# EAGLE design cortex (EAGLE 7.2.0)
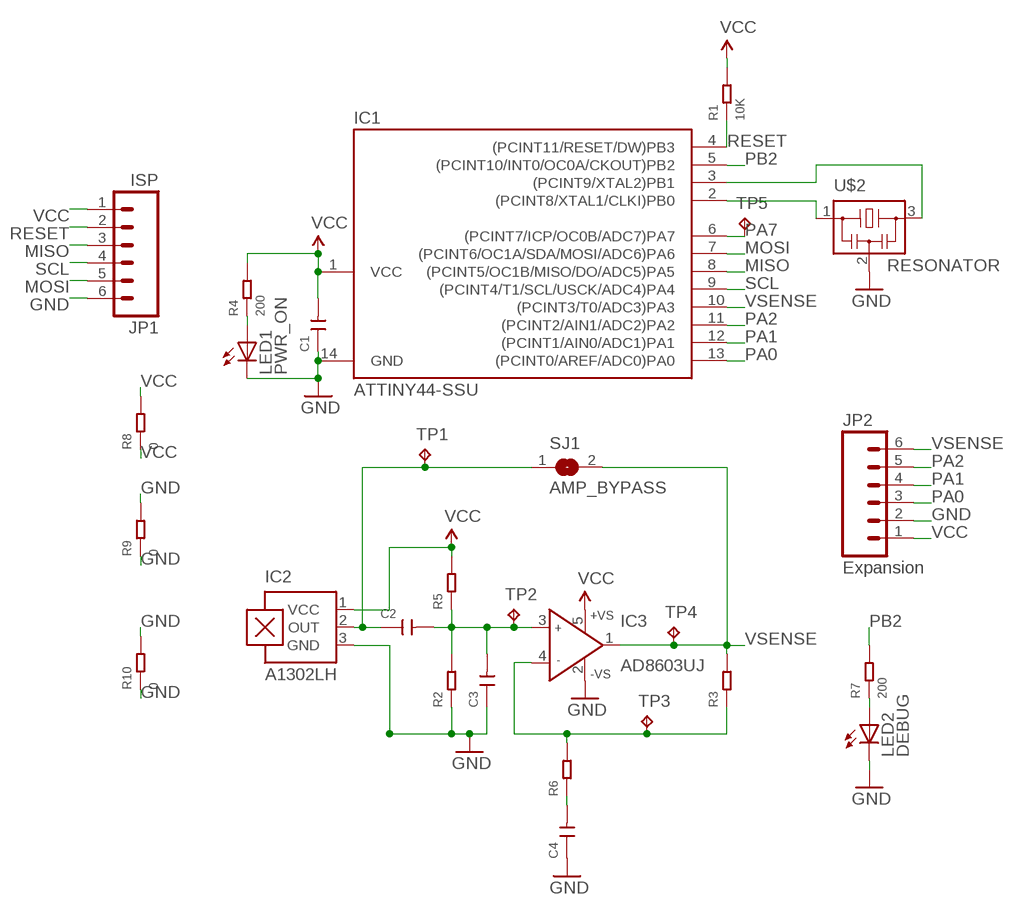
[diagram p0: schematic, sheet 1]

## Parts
C1  CAP-0805  [C0805]
C2  CAP-0805  [C0805]
C3  CAP-0805  [C0805]
C4  CAP-0805  [C0805]
IC1  ATTINY44-SSU  [SOIC14]
IC2  A1302LH  [SOT23-W]
IC3  AD8603UJ  [SOT23-5]
JP1  ISP  M06SMD-FEMALE-V2  [1X06-SMD-FEMALE-V2]
JP2  Expansion  M06SMD-FEMALE-V2  [1X06-SMD-FEMALE-V2]
LED1  PWR_ON  LEDCHIPLED_0805  [CHIPLED_0805]
LED2  DEBUG  LEDCHIPLED_0805  [CHIPLED_0805]
R1  10K  RES-0805  [R0805]
R2  RES-0805  [R0805]
R3  RES-0805  [R0805]
R4  200  RES-0805  [R0805]
R5  RES-0805  [R0805]
R6  RES-0805  [R0805]
R7  200  RES-0805  [R0805]
R8  0  RES-1206  [R1206]
R9  0  RES-1206  [R1206]
R10  0  RES-1206  [R1206]
SJ1  AMP_BYPASS  SJ  [SJ]
TP1  TPTP15R  [TP15R]
TP2  TPTP15R  [TP15R]
TP3  TPTP15R  [TP15R]
TP4  TPTP15R  [TP15R]
TP5  TPTP15R  [TP15R]
U$2  RESONATOR  [EFOBM]

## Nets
GND: C1.1 C3.1 C4.1 IC1.14(GND) IC2.3(GND) IC3.2(-VS) JP1.6 JP2.2 LED1.C LED2.C R2.1 R9.1 R9.2 R10.1 R10.2 U$2.2
HALL_VOUT: C2.1 IC2.2(OUT) SJ1.1 TP1.TP
MISO: IC1.8((PCINT5/OC1B/MISO/DO/ADC5)PA5) JP1.3
MOSI: IC1.7((PCINT6/OC1A/SDA/MOSI/ADC6)PA6) JP1.5
N$1: IC1.2((PCINT8/XTAL1/CLKI)PB0) U$2.1
N$2: IC1.3((PCINT9/XTAL2)PB1) U$2.3
N$3: IC3.4(IN-) R3.1 R6.2 TP3.TP
N$4: C4.2 R6.1
N$5: LED1.A R4.1
N$6: C2.2 C3.2 IC3.3(IN+) R2.2 R5.1 TP2.TP
N$7: LED2.A R7.1
PA0: IC1.13((PCINT0/AREF/ADC0)PA0) JP2.3
PA1: IC1.12((PCINT1/AIN0/ADC1)PA1) JP2.4
PA2: IC1.11((PCINT2/AIN1/ADC2)PA2) JP2.5
PA7: IC1.6((PCINT7/ICP/OC0B/ADC7)PA7) TP5.TP
PB2: IC1.5((PCINT10/INT0/OC0A/CKOUT)PB2) R7.2
RESET: IC1.4((PCINT11/RESET/DW)PB3) JP1.2 R1.1
SCL: IC1.9((PCINT4/T1/SCL/USCK/ADC4)PA4) JP1.4
VCC: C1.2 IC1.1(VCC) IC2.1(VCC) IC3.5(+VS) JP1.1 JP2.1 R1.2 R4.2 R5.2 R8.1 R8.2
VSENSE: IC1.10((PCINT3/T0/ADC3)PA3) IC3.1(OUT) JP2.6 R3.2 SJ1.2 TP4.TP

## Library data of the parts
C1-C4 = Discrete:CAP: Ceramic Capacitors
IC1 = fab:ATTINY44
IC2 = allegro:A13*?: Linear Hall Effect Sensor ICs Continuous-Time Ratiometric High-Temperature Operation Programmable Linear with Analog Output A1302 -Replacement- UGN3503 Source: http://www.allegromicro.com/en/Products/Part_Numbers/1301/1301.pdf http://www.allegromicro.com/en/Products/Part_Numbers/1321/1321.pdf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; MF: ALLEGRO MICROSYSTEMS, INC.; MPN: A1302ELHLT-T; OC_FARNELL: 1457209; OC_NEWARK: 31K6638
IC3 = analog-devices:AD8603: Precision Micropower, Low Noise CMOS, Rail-to-Rail Input/Output Operational Amplifiers Source: http://www.analog.com/static/imported-files/data_sheets/AD8603_8607_8609.pdf; MF: ALTERA CORPORATION; MPN: AD8603AUJZ-REEL7; OC_FARNELL: 1651290; OC_NEWARK: 59K6904
JP1 JP2 = SparkFun-Connectors:M06: Header 6 Standard 6-pin 0.1" header. Use with straight break away headers (SKU : PRT-00116), right angle break away headers (PRT-00553), swiss pins (PRT-00743), machine pins (PRT-00117), and female headers (PRT-00115). Molex polarized connector foot print use with SKU : PRT-08094 with associated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
LED1 LED2 = led:LED: LED
R1-R10 = Discrete:RES
SJ1 = jumper:SJ: SMD solder JUMPER
TP1-TP5 = testpad:TP: Test pad
U$2 = fab:RESONATOR

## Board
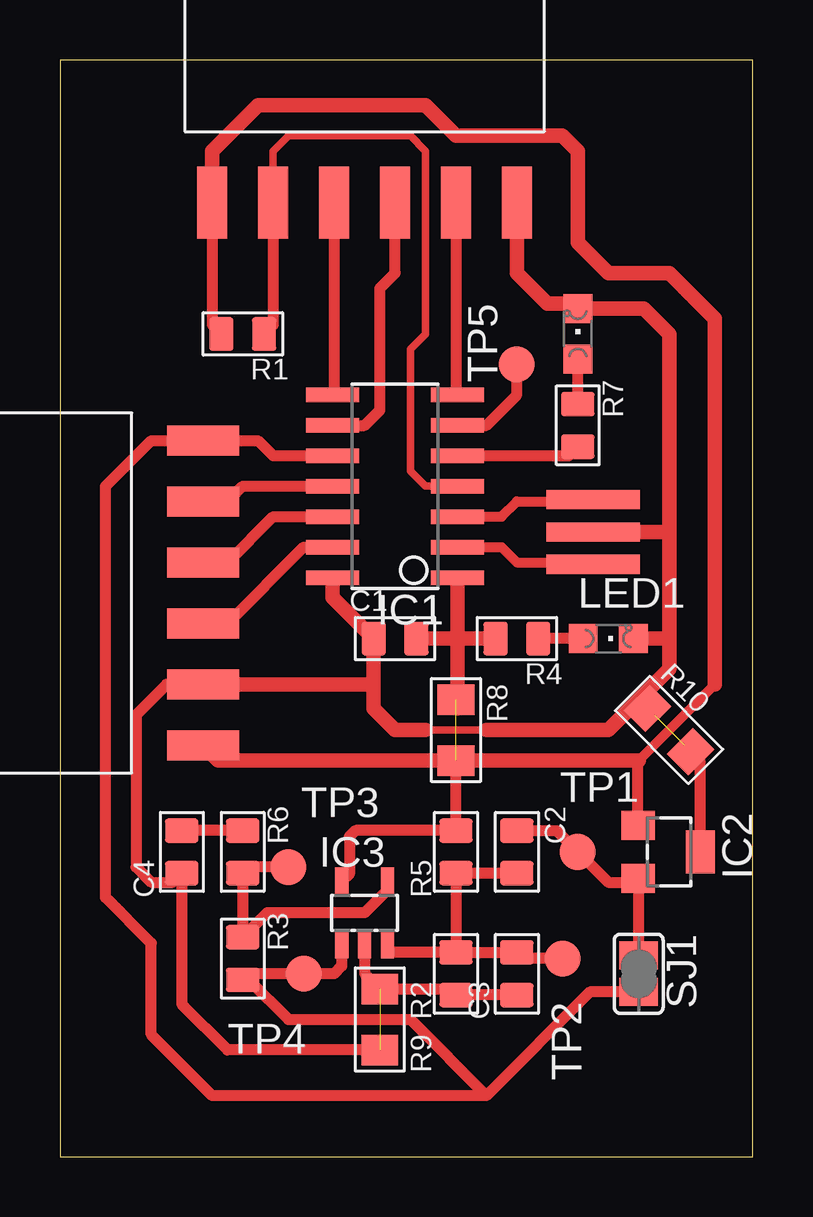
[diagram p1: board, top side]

Size 28.88 x 45.71 mm. Coordinates in mm from the lower left corner, seen from the top.
Outline: 0,0 28.88,0 28.88,45.71 0,45.71 0,0
Copper layers (1*16): Top 0.035mm / dielectric 1.5mm / Bottom 0.035mm
Design rules "fab_1_64_mil *": minimum track width 10mil, minimum drill 24mil, track to track 16mil, track to pad 14mil, pad to pad 14mil, via to via 14mil, smd to smd 14mil, copper to edge 40mil, drill to drill 8mil, minimum pad ring 10mil, minimum via ring 8mil, stop-mask expansion 4mil, vias tented up to drill 0mil, thermal gap 10mil

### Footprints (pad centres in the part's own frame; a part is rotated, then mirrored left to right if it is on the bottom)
C0805 = smd 1.016 x 1.397: 1 -0.889,0; 2 0.889,0
SOIC14 = smd 0.61 x 2.21: 1 -3.81,-2.603; 2 -2.54,-2.603; 3 -1.27,-2.603; 4 0,-2.603; 5 1.27,-2.603; 6 2.54,-2.603; 7 3.81,-2.603; 8 3.81,2.603; 9 2.54,2.603; 10 1.27,2.603; 11 0,2.603; 12 -1.27,2.603; 13 -2.54,2.603; 14 -3.81,2.603
SOT23-W = smd 1.2 x 1.4: 1 -1.1,-1.3; 2 1.1,-1.3 | smd 1.8 x 1.2: 3 0,1.3
SOT23-5 = smd 0.55 x 1.2: 1 -0.95,-1.3; 2 0,-1.3; 3 0.95,-1.3; 4 0.95,1.3; 5 -0.95,1.3
1X06-SMD-FEMALE-V2 = smd 1.25 x 3: 1 6.35,3.425; 2 3.81,3.425; 3 1.27,3.425; 4 -1.27,3.425; 5 -3.81,3.425; 6 -6.35,3.425
CHIPLED_0805 = smd 1.2 x 1.2: A 0,-1.05; C 0,1.05
R0805 = smd 1.397 x 1.016: 1 0,0.889; 2 0,-0.889
R1206 = smd 1.27 x 1.524: 1 -1.27,0; 2 1.27,0
SJ = smd 1.168 x 1.6: 1 -0.762,0; 2 0.762,0
TP15R = smd 1.5 x 1.5: TP 0,0
EFOBM = smd 0.8 x 3.9: 1 -1.35,0; 2 0,0; 3 1.35,0

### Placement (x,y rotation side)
C1  13.97,21.59 0 top
C2  19.05,12.7 270 top
C3  19.05,7.62 90 top
C4  5.08,12.7 90 top
IC1  13.97,27.94 90 top
IC2  25.4,12.7 270 top
IC3  12.7,10.16 0 top
JP1  12.7,43.18 180 top
JP2  2.54,23.49 270 top
LED1  22.86,21.59 270 top
LED2  21.59,34.29 0 top
R1  7.62,34.29 270 top
R2  16.51,7.62 180 top
R3  7.62,8.25 0 top
R4  19.05,21.59 270 top
R5  16.51,12.7 180 top
R6  7.62,12.7 0 top
R7  21.59,30.48 0 top
R8  16.51,17.78 270 top
R9  13.33,5.71 270 top
R10  25.4,17.78 315 top
SJ1  24.13,7.62 270 top
TP1  21.59,12.7 270 top
TP2  20.95,8.25 270 top
TP3  9.53,12.06 180 top
TP4  10.16,7.62 180 top
TP5  19.05,33.02 90 top
U$2  22.23,26.04 90 top

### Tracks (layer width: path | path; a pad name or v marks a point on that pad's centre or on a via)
GND  (2 unrouted)
  Top 0.305: 15.24,17.78 17.78,17.78
  Top 0.457: C3.1 R2.1 16.26,6.98 R9.1 12.7,7.62 IC3.2 | JP2.2 4.44,19.69 3.17,18.41 3.17,12.06 3.81,11.43 4.7,11.43 C4.1 5.08,6.35 6.99,4.45 R9.2 | 26.67,12.67 IC2.3 26.67,12.73 26.67,16.51 26.03,17.15 R10.2 | R10.1 24.77,18.41 24.13,19.05
  Top 0.61: IC1.14 11.37,23.3 C1.1 13.08,19.69 | JP1.6 19.05,36.83 20.32,35.56 21.37,35.56 LED2.C 24.35,35.34 25.4,34.29 25.4,26.04 | 25.4,26.04 25.4,21.59 | 25.4,21.59 25.4,20.32 24.13,19.05 22.86,17.78 17.78,17.78 | U$2.2 25.4,26.04 | LED1.C 25.4,21.59 | 15.24,17.78 13.97,17.78 13.08,18.67 13.08,19.69 | JP2.2 13.08,19.69
HALL_VOUT
  Top 0.457: C2.1 20.7,13.59 TP1.TP 22.86,11.43 23.93,11.43 IC2.2 24.13,11.57 SJ1.1
MISO
  Top 0.457: JP1.3 11.43,31.81 IC1.8
MOSI
  Top 0.457: JP1.5 16.51,31.81 IC1.7
N$1
  Top 0.406: IC1.2 18.41,25.4 19.05,24.77 23.41,24.77 U$2.1
N$2
  Top 0.406: IC1.3 18.41,26.67 19.05,27.3 23.41,27.3 U$2.3
N$3
  Top 0.457: IC3.4 13.65,11.11 12.7,10.16 8.64,10.16 R3.1 R6.2 7.62,12.06 TP3.TP
N$4
  Top 0.457: R6.1 C4.2
N$5
  Top 0.457: LED1.A R4.1
N$6
  Top 0.457: C2.2 R5.1 R2.2 | R2.2 C3.2 19.3,8.25 TP2.TP | R2.2 13.65,8.51 IC3.3
N$7
  Top 0.457: R7.1 LED2.A
PA0
  Top 0.457: JP2.3 6.99,22.23 10.16,25.4 IC1.13
PA1
  Top 0.457: JP2.4 6.99,24.77 8.89,26.67 IC1.12
PA2
  Top 0.457: JP2.5 6.99,27.3 7.62,27.94 IC1.11
PA7
  Top 0.457: IC1.6 17.78,30.48 19.05,31.75 TP5.TP
PB2
  Top 0.457: IC1.5 21.21,29.21 R7.2
RESET
  Top 0.305: JP1.2 8.89,41.91 9.53,42.55 14.6,42.55 15.24,41.91 15.24,34.29 14.6,33.66 14.6,28.58 15.24,27.94 IC1.4
  Top 0.457: JP1.2 8.89,34.67 R1.1
SCL
  Top 0.457: IC1.9 12.7,30.48 13.33,31.12 13.33,36.2 13.97,36.83 JP1.4
VCC  (1 unrouted)
  Top 0.406: 27.3,19.69 24.13,16.51
  Top 0.457: 16.57,23.3 16.57,23.18 | JP1.1 6.35,34.67 R1.2 | IC3.5 12.06,11.77 12.06,13.34 12.32,13.59 R5.2 R8.2 | IC2.1 24.1,16.48 24.13,16.51
  Top 0.61: 16.57,23.3 IC1.1 16.57,21.59 | R8.1 16.57,18.67 16.57,21.59 | R4.2 16.57,21.59 | 16.57,21.59 C1.2 | JP1.1 6.35,41.91 8.26,43.81 15.24,43.81 16.51,42.55 20.95,42.55 21.59,41.91 21.59,38.1 22.86,36.83 25.4,36.83 27.3,34.92 27.3,19.69 | 24.13,16.51 R8.2 6.6,16.51 JP2.1 6.22,16.89
VSENSE
  Top 0.457: IC1.10 8.89,29.21 8.26,29.84 JP2.6 3.81,29.84 1.9,27.94 1.9,10.8 3.81,8.89 3.81,5.08 6.35,2.54 17.78,2.54 | SJ1.2 22.1,6.86 17.78,2.54 | IC3.1 11.75,7.94 11.43,7.62 TP4.TP 7.87,7.62 R3.2 7.87,7.37 9.53,5.71 14.6,5.71 17.78,2.54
